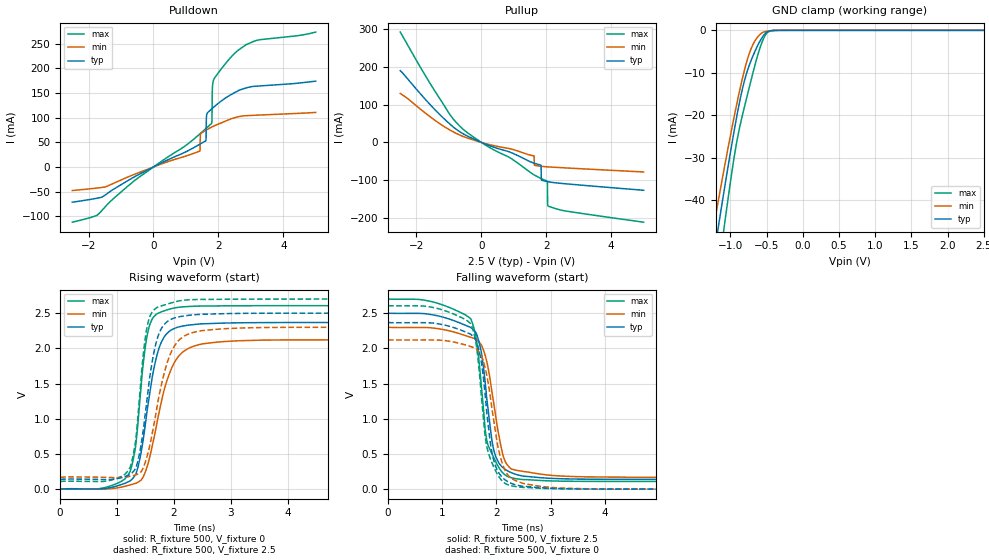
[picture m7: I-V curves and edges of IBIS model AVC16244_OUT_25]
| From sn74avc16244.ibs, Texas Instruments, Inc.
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[Model]   AVC16244_OUT_25
Model_type  3-state
Enable   Active-Low
Vref =   0
Rref =   500
Cref =   30p
Vmeas =   1.25
| variable   typ   min   max
C_comp   4.24pF   3.29pF   5.19pF
| C_pullup   8.00pF   0.77pF   28.20pF
| C_pulldown   14.46pF   1.93pF   42.49pF
| C_tri-state   4.24pF   3.29pF   5.19pF
[Temperature Range]   40   100   -40
| Ambient temperature   25   85   -40
[Voltage range]   2.5   2.3   2.7
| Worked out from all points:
|   slope of the pulldown table from 0 to 0.375 V, typ, clamps not added: 30.4 ohm
|   slope of the pullup table from 0 to 0.375 V, typ, clamps not added: 30.1 ohm
|   GND clamp passes 1 mA (typ) near -0.53 V on its own axis
|   rising waveform, R_fixture 500, V_fixture 0: 20-80 % time 288ps typ, 384ps min, 201ps max; typ from 0 V to 2.37 V
|   falling waveform, R_fixture 500, V_fixture 2.5: 20-80 % time 238ps typ, 286ps min, 228ps max; typ from 2.5 V to 0.139 V
|   rising waveform, R_fixture 500, V_fixture 2.5: 20-80 % time 253ps typ, 348ps min, 187ps max; typ from 0.139 V to 2.5 V
|   falling waveform, R_fixture 500, V_fixture 0: 20-80 % time 229ps typ, 285ps min, 231ps max; typ from 2.37 V to 0 V
[GND Clamp]
| AVC16244_OUT_25
|   Voltage   I(typ)   I(min)   I(max)
-2.5V     -203.1mA   -176.6mA   -245mA
-1.25V    -55.32mA   -47.91mA   -67.57mA
-1.22V    -52.01mA   -45.03mA   -63.58mA
-1.16V    -45.45mA   -39.32mA   -55.68mA
-1.08V    -36.9mA    -31.89mA   -45.41mA
-935mV    -22.33mA   -19.15mA   -28.4mA
-815mV    -12.4mA    -9.921mA   -18.58mA
-695mV    -6.258mA   -3.551mA   -10.39mA
-550mV    -1.377mA   -457.5uA   -2.217mA
-490mV    -343uA     -178.6uA   -509.8uA
-380mV    -18.7uA    -25.17uA   -12.35uA
2.5V      974.5pA    11.59nA    39.78pA
[Pulldown]
| AVC16244_OUT_25
|   Voltage   I(typ)   I(min)   I(max)
-2.5V     -71.56mA   -47.84mA   -112.1mA
-1.73V    -63.38mA   -42.71mA   -97.81mA
1.425V    46.07mA    32.15mA    66.84mA
1.455V    47.21mA    67.92mA    68.59mA
1.61V     53.02mA    74.39mA    77.73mA
1.64V     105.9mA    75.53mA    79.51mA
1.79V     117.7mA    80.88mA    88.21mA
1.805V    118.5mA    81.38mA    100.8mA
1.815V    119.1mA    81.71mA    160.3mA
1.855V    121.4mA    83mA       176.9mA
2.615V    154.9mA    102mA      237.2mA
5V        174.3mA    110.8mA    274mA
[Pullup]
| AVC16244_OUT_25
|   Voltage   I(typ)   I(min)   I(max)
-2.5V     190.4mA    129.9mA    292.9mA
-845mV    39.51mA    27.08mA    59.91mA
1.62V     -54.9mA    -35.73mA   -85.82mA
1.635V    -55.33mA   -60.76mA   -86.58mA
1.83V     -60.18mA   -63.23mA   -95.41mA
1.84V     -61.44mA   -63.34mA   -95.82mA
1.85V     -100mA     -63.44mA   -96.22mA
2.025V    -103.7mA   -64.84mA   -102.8mA
2.035V    -103.9mA   -64.9mA    -106.3mA
2.04V     -104mA     -64.93mA   -160.9mA
2.06V     -104.3mA   -65.04mA   -169.3mA
5V        -127mA     -78.45mA   -211.8mA
[Ramp]
| AVC16244_OUT_25
| variable   typ   min   max
dV/dt_r   1.42/2.95E-10   1.27/3.91E-10   1.56/2.08E-10
dV/dt_f   1.42/2.54E-10   1.28/2.93E-10   1.55/2.40E-10
R_load = 500
[Rising Waveform]
| AVC16244_OUT_25
R_fixture =   500
C_fixture =   0
L_fixture =   0
V_fixture =   0
V_fixture_min = 0
V_fixture_max = 0
|   Time   V(typ)   V(min)   V(max)
0s        25.65nV    106.5nV    1.147nV
1.195ns   103mV      52.45mV    203mV
1.305ns   181.7mV    77.03mV    504.7mV
1.375ns   334.8mV    101.6mV    1.002V
1.475ns   780.5mV    200.5mV    1.877V
1.575ns   1.357V     451.8mV    2.331V
1.785ns   2.096V     1.258V     2.52V
2.15ns    2.316V     1.943V     2.589V
3.92ns    2.366V     2.12V      2.606V
34.99ns   2.367V     2.122V     2.606V
[Falling Waveform]
| AVC16244_OUT_25
R_fixture =   500
C_fixture =   0
L_fixture =   0
V_fixture =   2.5
V_fixture_min = 2.3
V_fixture_max = 2.7
|   Time   V(typ)   V(min)   V(max)
0s        2.5V       2.3V       2.7V
1.525ns   2.296V     2.157V     2.419V
1.625ns   2.216V     2.13V      2.142V
1.71ns    1.985V     2.06V      1.559V
1.79ns    1.526V     1.903V     856.4mV
1.845ns   1.133V     1.724V     623.3mV
1.96ns    527mV      1.169V     431mV
2.135ns   296.4mV    446.9mV    217.7mV
2.48ns    187.1mV    253.7mV    137.1mV
34.99ns   138.6mV    167.6mV    109.3mV
[Rising Waveform]
| AVC16244_OUT_25
R_fixture =   500
C_fixture =   0
L_fixture =   0
V_fixture =   2.5
V_fixture_min = 2.3
V_fixture_max = 2.7
|   Time   V(typ)   V(min)   V(max)
0s        138.6mV    167.6mV    109.3mV
1.045ns   156.6mV    164.5mV    168.8mV
1.23ns    206.9mV    183mV      307.5mV
1.31ns    273.5mV    197.8mV    595.9mV
1.47ns    890.7mV    319.7mV    1.969V
1.57ns    1.554V     598.9mV    2.435V
1.785ns   2.287V     1.496V     2.604V
1.965ns   2.417V     1.967V     2.648V
2.19ns    2.462V     2.178V     2.685V
34.99ns   2.5V       2.3V       2.7V
[Falling Waveform]
| AVC16244_OUT_25
R_fixture =   500
C_fixture =   0
L_fixture =   0
V_fixture =   0
V_fixture_min = 0
V_fixture_max = 0
|   Time   V(typ)   V(min)   V(max)
0s        2.367V     2.122V     2.606V
1.525ns   2.2V       2.026V     2.351V
1.625ns   2.111V     1.995V     2.062V
1.715ns   1.832V     1.907V     1.375V
1.79ns    1.35V      1.726V     760.1mV
1.87ns    761.9mV    1.399V     469.7mV
1.97ns    356.6mV    874.3mV    282.3mV
2.12ns    158mV      338.5mV    105mV
2.47ns    42.73mV    87mV       26.46mV
34.99ns   32.36nV    139.9nV    -11.47nV
